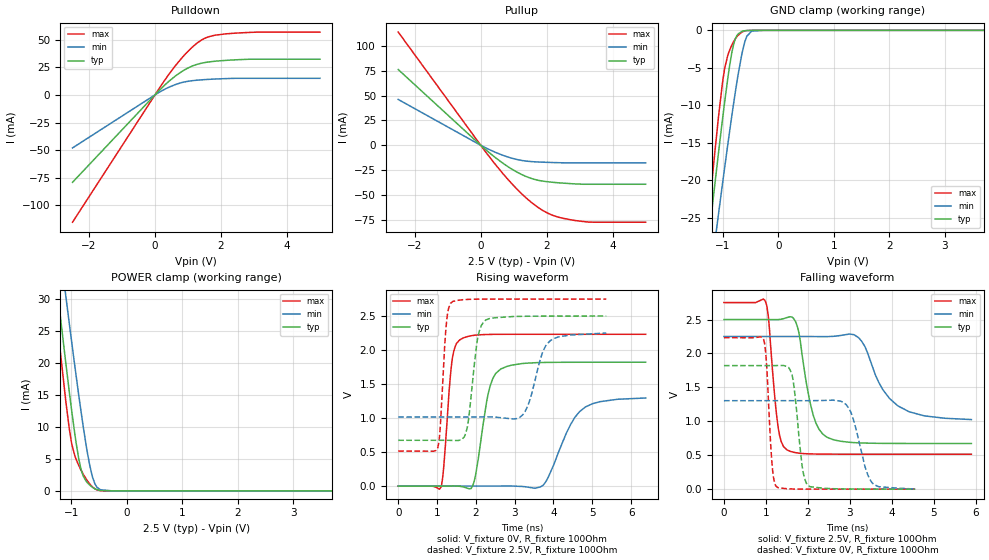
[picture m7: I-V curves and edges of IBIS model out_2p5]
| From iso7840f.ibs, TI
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|   out_2p5 Model
[Model]   out_2p5
Model_type   3-state
Polarity   Non-Inverting
Vmeas = 1.25
Vref = 0
Cref = 15pF
Rref = 150
|   typ   min   max
|   (nom PVT)   (fast PVT)   (slow PVT)
C_comp   1.027e-12   9.377e-13   1.105e-12
| Where nom  PVT is Nominal Process, 2.5V, 27C
|   Fast PVT is Strong Process,  2.75V, -55C
|   Slow PVT is Weak Process,   2.25V, 150C
[Voltage Range]   2.5   2.25   2.75
|Junction Temperature
[Temperature Range]   27   150   -55
[Pullup Reference]   2.5   2.25   2.75
[Pulldown Reference]   0   0   0
[Power Clamp Reference]   2.5   2.25   2.75
[GND Clamp Reference]   0   0   0
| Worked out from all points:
|   slope of the pulldown table from 0 to 0.375 V, typ, clamps not added: 34 ohm
|   slope of the pullup table from 0 to 0.375 V, typ, clamps not added: 35.4 ohm
|   GND clamp passes 1 mA (typ) near -0.76 V on its own axis
|   POWER clamp passes 1 mA (typ) near -0.68 V on its own axis
|   falling waveform, V_fixture 2.5V, R_fixture 100Ohm: 20-80 % time 326ps typ, 642ps min, 190ps max; typ from 2.5 V to 0.673 V
|   rising waveform, V_fixture 0V, R_fixture 100Ohm: 20-80 % time 310ps typ, 623ps min, 179ps max; typ from 0 V to 1.82 V
|   rising waveform, V_fixture 2.5V, R_fixture 100Ohm: 20-80 % time 211ps typ, 359ps min, 135ps max; typ from 0.673 V to 2.5 V
|   falling waveform, V_fixture 0V, R_fixture 100Ohm: 20-80 % time 179ps typ, 324ps min, 116ps max; typ from 1.82 V to 0 V
[Pulldown]
|   Voltage   I(typ)   I(min)   I(max)
-2.5V     -79.05mA   -47.97mA   -115.1mA
242.5mV   7.369mA    4.254mA    10.99mA
604.8mV   16.75mA    9.164mA    25.83mA
786.3mV   20.6mA     10.9mA     32.43mA
1.1V      25.7mA     12.7mA     42.29mA
1.292V    27.74mA    13.31mA    47.16mA
1.408V    28.6mA     13.59mA    49.53mA
1.631V    29.75mA    14.02mA    52.54mA
2.148V    31.19mA    14.7mA     55.16mA
3.105V    32.21mA    14.98mA    56.72mA
5V        32.21mA    14.98mA    56.75mA
[GND Clamp]
|   Voltage   I(typ)   I(min)   I(max)
-2.5V     -113.8mA   -109.3mA   -126.7mA
-1.327V   -32.82mA   -39.06mA   -30.54mA
-1.16V    -21.76mA   -29.34mA   -17.63mA
-1.073V   -16.17mA   -24.36mA   -11.36mA
-960mV    -9.309mA   -18.06mA   -4.938mA
-871mV    -4.546mA   -13.26mA   -2.575mA
-805mV    -1.936mA   -9.853mA   -1.543mA
-742.5mV  -678.4uA   -6.825mA   -835.1uA
-655mV    -148uA     -3.167mA   -231.5uA
-565mV    -24.88uA   -787.3uA   -32.49uA
-475mV    -3.219uA   -94.87uA   -2.89uA
5V        0A         0A         0A
[Pullup]
|   Voltage   I(typ)   I(min)   I(max)
-2.5V     76.08mA    46.03mA    113.8mA
0V        0A         0A         0A
350.8mV   -9.946mA   -5.734mA   -15.38mA
665mV     -17.88mA   -10.02mA   -28.2mA
1.061V    -26.29mA   -14.04mA   -42.81mA
1.343V    -30.95mA   -15.79mA   -51.94mA
1.605V    -34.09mA   -16.59mA   -59.28mA
1.905V    -36.18mA   -17.06mA   -66.05mA
2.148V    -37.13mA   -17.34mA   -70mA
2.754V    -38.65mA   -17.71mA   -75.11mA
3.3V      -39.22mA   -17.71mA   -77.31mA
5V        -39.22mA   -17.71mA   -77.36mA
[POWER Clamp]
|   Voltage   I(typ)   I(min)   I(max)
-2.5V     130.5mA    131.5mA    137.5mA
-1.331V   37.45mA    46.69mA    32.98mA
-1.194V   27mA       37.02mA    21.48mA
-1.096V   19.79mA    30.25mA    13.84mA
-984.8mV  12.01mA    22.71mA    7.082mA
-912.5mV  7.491mA    17.96mA    4.93mA
-833.5mV  3.695mA    12.97mA    3.404mA
-782.5mV  2.286mA    9.916mA    2.578mA
-667.5mV  905.1uA    3.994mA    1.088mA
-539.3mV  198.3uA    596.8uA    170.5uA
-250mV    142.1nA    1.582uA    12.72nA
5V        0A         0A         0A
[Ramp]
R_load = 100
|   typ   min   max
dV/dt_r   1.09259/3.08138e-10   0.773097/6e-10   1.33922/1.77917e-10
dV/dt_f   1.09612/3.23289e-10   0.734486/6.3101e-10   1.34089/1.89259e-10
[Falling Waveform]
V_fixture = 2.5V
V_fixture_min = 2.25V
V_fixture_max = 2.75V
R_fixture = 100Ohm
|   Time   V(typ)   V(min)   V(max)
0s        2.5V       2.25V      2.75V
990ps     2.5V       2.25V      2.764V
1.288ns   2.499V     2.25V      932.3mV
1.502ns   2.529V     2.25V      579.3mV
1.748ns   2.401V     2.25V      534.2mV
2.124ns   1.101V     2.25V      518.7mV
2.438ns   773.7mV    2.248V     516.2mV
3.206ns   682.8mV    2.235V     515.2mV
4.152ns   673.9mV    1.226V     515.2mV
5.9ns     673.1mV    1.026V     515.2mV
[Rising Waveform]
V_fixture = 0V
V_fixture_min = 0V
V_fixture_max = 0V
R_fixture = 100Ohm
|   Time   V(typ)   V(min)   V(max)
0s        2.759nV    92.09nV    1.558nV
1.106ns   -50.52uV   -598.6pV   -11.27mV
1.378ns   985.1uV    1.177uV    1.808V
1.582ns   -2.948mV   3.582uV    2.149V
1.924ns   12.2mV     -18.45uV   2.215V
2.316ns   1.353V     6.248uV    2.229V
2.644ns   1.722V     808.8uV    2.232V
3.728ns   1.817V     8.286mV    2.232V
4.822ns   1.821V     1.163V     2.232V
6.376ns   1.821V     1.295V     2.232V
[Rising Waveform]
V_fixture = 2.5V
V_fixture_min = 2.25V
V_fixture_max = 2.75V
R_fixture = 100Ohm
|   Time   V(typ)   V(min)   V(max)
0s        673.1mV    1.016V     515.1mV
1.016ns   673.1mV    1.016V     558.3mV
1.246ns   673.2mV    1.016V     2.422V
1.404ns   670.5mV    1.016V     2.715V
1.74ns    779.2mV    1.016V     2.743V
2.048ns   2.178V     1.016V     2.748V
2.256ns   2.441V     1.017V     2.749V
3.212ns   2.496V     1.05V      2.75V
3.918ns   2.499V     2.139V     2.75V
5.36ns    2.5V       2.25V      2.75V
[Falling Waveform]
V_fixture = 0V
V_fixture_min = 0V
V_fixture_max = 0V
R_fixture = 100Ohm
|   Time   V(typ)   V(min)   V(max)
0s        1.821V     1.304V     2.232V
944ps     1.821V     1.304V     2.208V
1.154ns   1.821V     1.304V     315.2mV
1.28ns    1.822V     1.304V     24.79mV
1.624ns   1.688V     1.304V     2.768mV
1.864ns   342.3mV    1.304V     579.5uV
1.998ns   56.53mV    1.304V     257.4uV
2.916ns   3.114mV    1.245V     4.44uV
3.578ns   669uV      67.55mV    350.7nV
4.56ns    5.479uV    1.617mV    1.776nV
